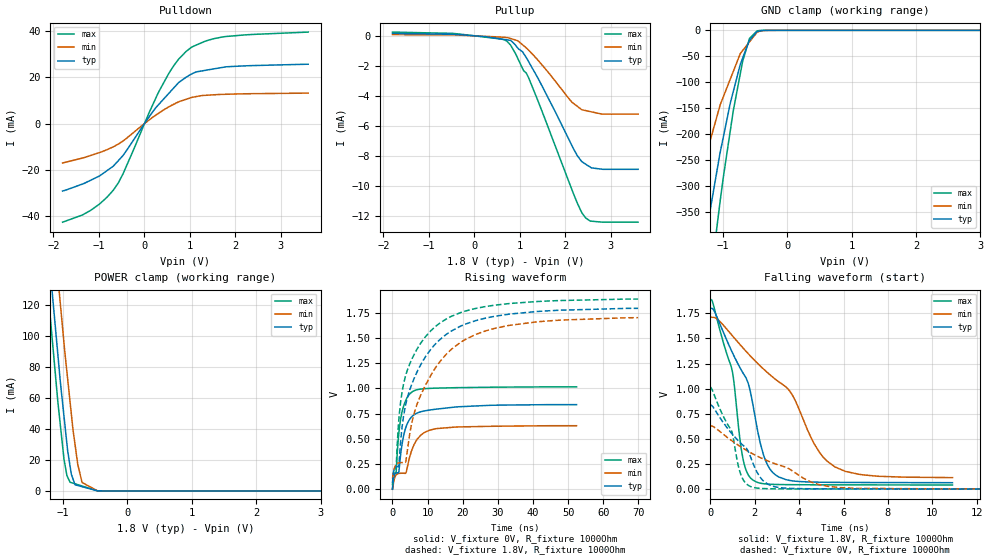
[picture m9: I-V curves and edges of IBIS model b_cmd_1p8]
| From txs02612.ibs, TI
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|   b_cmd_1p8 Model
[Model]   b_cmd_1p8
Model_type   I/O
Polarity   Non-Inverting
Enable   Active-High
Vinl = 0.15
Vinh = 1.6
Vmeas = 0.9
Vref = 0.9
Cref = 2pF
Rref = 1000
|   typ   min   max
|   (nom PVT)   (fast PVT)   (slow PVT)
|C_comp from frequency sweep method (F=30MHz)
C_comp   9.470e-12   9.412e-12   9.537e-12
|ON state : BUFFER OUTPUT TURNED HIGH
|C_comp   9.284e-12   9.057e-12   9.650e-12
|OFF state: BUFFER IN HIGH IMPEDANCE
|C_comp   9.470e-12   9.412e-12   9.537e-12
|C_comp from LC tank measurement(L=1nH)
|Average
|Resonant Frequency(Hz)   1.720e+09   1.725e+09   1.720e+09
|C_comp   8.571e-12   8.521e-12   8.571e-12
|ON state : BUFFER OUTPUT TURNED HIGH
|Resonant Frequency(Hz)   1.720e+09   1.730e+09   1.720e+09
|C_comp   8.571e-12   8.472e-12   8.571e-12
|OFF state: BUFFER IN HIGH IMPEDANCE
|Resonant Frequency(Hz)   1.720e+09   1.720e+09   1.720e+09
|C_comp   8.571e-12   8.571e-12   8.571e-12
[Model spec]
|subparameter
Vinl   0.15   0.15   0.15
Vinh   1.6   1.51   1.69
| Where nom  PVT is Nominal Process, 1.8V, 27C
|   Fast PVT is Strong Process,  1.89V, -40C
|   Slow PVT is Weak Process,   1.71V, 125C
[Voltage Range]   1.8   1.71   1.89
|Ambient Temperature   25   85   -40
|Junction Temperature
[Temperature Range]   27   125   -40
[Pullup Reference]   1.8   1.71   1.89
[Pulldown Reference]   0   0   0
[Power Clamp Reference]   1.8   1.71   1.89
[GND Clamp Reference]   0   0   0
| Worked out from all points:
|   slope of the pulldown table from 0 to 0.27 V, typ, clamps not added: 36.7 ohm
|   slope of the pullup table from 0 to 0.27 V, typ, clamps not added: 3.97 kohm
|   GND clamp passes 1 mA (typ) near -0.41 V on its own axis
|   POWER clamp passes 1 mA (typ) near -0.55 V on its own axis
|   falling waveform, V_fixture 1.8V, R_fixture 1000Ohm: 20-80 % time 1.51ns typ, 3.19ns min, 877ps max; typ from 1.8 V to 0.067 V
|   rising waveform, V_fixture 0V, R_fixture 1000Ohm: 20-80 % time 2.73ns typ, 6.45ns min, 1.97ns max; typ from 0.002 V to 0.839 V
|   rising waveform, V_fixture 1.8V, R_fixture 1000Ohm: 20-80 % time 10.2ns typ, 12.2ns min, 8.18ns max; typ from 0.062 V to 1.79 V
|   falling waveform, V_fixture 0V, R_fixture 1000Ohm: 20-80 % time 1.55ns typ, 3.23ns min, 887ps max; typ from 0.841 V to 0.004 V
[Pulldown]
|   Voltage   I(typ)   I(min)   I(max)
-1.8V     -29.32mA   -17.13mA   -42.85mA
-1.181V   -24.61mA   -13.86mA   -37.7mA
-982.8mV  -22.71mA   -12.58mA   -34.86mA
-684.2mV  -18.49mA   -10.1mA    -28.94mA
-470.6mV  -13.87mA   -7.571mA   -21.83mA
91.8mV    2.61mA     1.386mA    4.229mA
332.6mV   8.71mA     4.758mA    14.46mA
655.8mV   15.72mA    8.499mA    25.46mA
1.015V    21.29mA    11.18mA    32.86mA
1.332V    23.09mA    12.25mA    35.75mA
1.727V    24.43mA    12.68mA    37.64mA
3.6V      25.77mA    13.22mA    39.72mA
[GND Clamp]
|   Voltage   I(typ)   I(min)   I(max)
-1.8V     -883.9mA   -527.4mA   -1.209A
-1.565V   -660.4mA   -397mA     -909.2mA
-1.353V   -470.2mA   -281.1mA   -656.2mA
-1.22V    -362mA     -222.3mA   -510.5mA
-1.168V   -324.5mA   -199.1mA   -453mA
-1.049V   -239.4mA   -146.5mA   -335mA
-885.6mV  -140.2mA   -93.88mA   -193.4mA
-839.2mV  -117.9mA   -79.22mA   -155mA
-691.7mV  -53.05mA   -38.74mA   -58.73mA
-585.9mV  -19.36mA   -22.04mA   -15.53mA
-470.6mV  -2.548mA   -3.851mA   -1.136mA
3.6V      0A         0A         0A
[Pullup]
|   Voltage   I(typ)   I(min)   I(max)
-1.8V     155.4uA    78.91uA    248.2uA
-470.6mV  103.1uA    57.99uA    162.5uA
712.5mV   -266.5uA   -117.2uA   -346.6uA
817.2mV   -354.7uA   -197uA     -724uA
1.083V    -1.171mA   -654.4uA   -2.32mA
1.139V    -1.436mA   -798.7uA   -2.471mA
1.461V    -3.181mA   -1.844mA   -4.813mA
2.153V    -7.36mA    -4.442mA   -10.31mA
2.368V    -8.389mA   -4.927mA   -11.81mA
2.548V    -8.742mA   -5.045mA   -12.33mA
2.808V    -8.882mA   -5.216mA   -12.4mA
3.6V      -8.888mA   -5.216mA   -12.41mA
[POWER Clamp]
|   Voltage   I(typ)   I(min)   I(max)
-1.8V     439.4mA    482.9mA    413.4mA
-1.232V   157.5mA    208.4mA    127.3mA
-1.154V   121.2mA    170.6mA    91.04mA
-1.044V   70.69mA    121.2mA    42.76mA
-984.7mV  47.41mA    94.63mA    20.01mA
-941.2mV  30.34mA    76.96mA    9.873mA
-892.1mV  15.92mA    57.46mA    5.603mA
-815.4mV  3.987mA    30.09mA    4.604mA
-772.9mV  3.509mA    17.2mA     4.05mA
-706.2mV  2.757mA    5.464mA    3.181mA
-470.3mV  111.6uA    136.8uA    109.5uA
3.6V      0A         0A         0A
[Ramp]
R_load = 1000
|   typ   min   max
dV/dt_r   0.503179/2.73307e-09   0.377901/6.4647e-09   0.608693/1.97124e-09
dV/dt_f   1.04274/1.50608e-09   0.961574/3.2023e-09   1.10934/8.78632e-10
[Falling Waveform]
V_fixture = 1.8V
V_fixture_min = 1.71V
V_fixture_max = 1.89V
R_fixture = 1000Ohm
|   Time   V(typ)   V(min)   V(max)
0s        1.8V       1.71V      1.89V
1ns       1.36V      1.527V     1.176V
1.475ns   1.158V     1.407V     310.9mV
1.9ns     874.9mV    1.305V     98.02mV
2.425ns   329.3mV    1.191V     56.66mV
3.1ns     123.3mV    1.067V     49.19mV
3.725ns   85.13mV    927.6mV    47.65mV
4.925ns   72.28mV    366.8mV    46.54mV
5.625ns   70.74mV    222.9mV    46.18mV
10.9ns    67.43mV    117.9mV    44.54mV
[Rising Waveform]
V_fixture = 0V
V_fixture_min = 0V
V_fixture_max = 0V
R_fixture = 1000Ohm
|   Time   V(typ)   V(min)   V(max)
0s        2.294mV    2.526mV    2.155mV
350ps     115.9mV    73.19mV    138.6mV
1.05ns    161.9mV    142.9mV    170.4mV
1.8ns     169.5mV    157.2mV    548.9mV
2.575ns   410.2mV    160mV      742.9mV
3.875ns   619.8mV    166.7mV    888.2mV
5.85ns    731.4mV    420.3mV    971.5mV
8.1ns     769.3mV    538.1mV    994.1mV
12.55ns   794.9mV    602.1mV    1.003V
52.4ns    839.5mV    630.6mV    1.016V
[Rising Waveform]
V_fixture = 1.8V
V_fixture_min = 1.71V
V_fixture_max = 1.89V
R_fixture = 1000Ohm
|   Time   V(typ)   V(min)   V(max)
0s        62.08mV    107.3mV    41.09mV
350ps     175.8mV    177.8mV    178.3mV
1.05ns    222.2mV    246.8mV    215.4mV
1.775ns   230mV      261.8mV    671.6mV
2.675ns   596.8mV    266mV      949.5mV
3.675ns   825.1mV    267.6mV    1.118V
6.65ns    1.138V     808.4mV    1.368V
12.83ns   1.462V     1.234V     1.63V
29.2ns    1.715V     1.596V     1.825V
69.9ns    1.793V     1.701V     1.885V
[Falling Waveform]
V_fixture = 0V
V_fixture_min = 0V
V_fixture_max = 0V
R_fixture = 1000Ohm
|   Time   V(typ)   V(min)   V(max)
0s        841mV      632.4mV    1.017V
975ps     555.6mV    484.3mV    576.4mV
1.25ns    488.6mV    442.2mV    254.6mV
1.425ns   449.9mV    417.2mV    125mV
2ns       223.5mV    344.8mV    17.97mV
2.375ns   89.86mV    304.8mV    9.441mV
2.875ns   29.36mV    259.1mV    6.736mV
4.65ns    7.056mV    65.41mV    5.247mV
5.85ns    6.205mV    18.73mV    4.947mV
22.32ns   3.703mV    4.634mV    3.169mV
